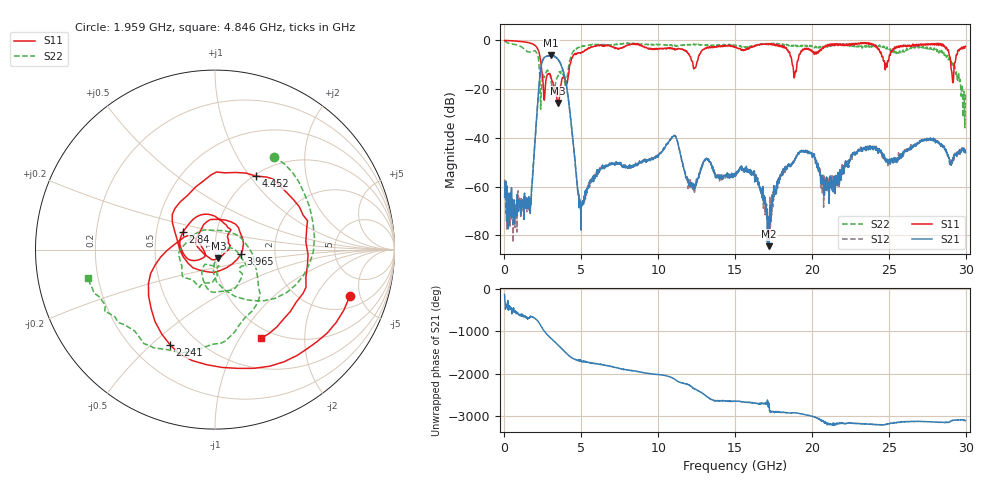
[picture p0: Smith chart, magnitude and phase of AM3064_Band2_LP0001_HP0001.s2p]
# Hz S DB R 50.0
!freq dBS11 angS11 dBS21 angS21 dBS12 angS12 dBS22 angS22
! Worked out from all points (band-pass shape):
!   1600 points, 10 MHz to 29.98 GHz, reference 50 ohm
!   highest |S21| = -6.21 dB at 3.046 GHz (marker M1); lowest = -84.5 dB at 17.22 GHz (marker M2)
!   |S21| within 3 dB of the highest: 2.436 GHz to 3.608 GHz (1.172 GHz wide, 38.8 % of centre)
!   lowest |S11| = -25.7 dB at 3.478 GHz (marker M3), VSWR 1.11, Z = 51.7 - j5.02 ohm
!   |S11| at or under -10 dB: 2.385 GHz to 4.259 GHz (1.874 GHz wide, 56.4 % of centre); 18.73 GHz to 19.02 GHz (292 MHz wide, 1.55 % of centre); 29.03 GHz to 29.26 GHz (229.2 MHz wide, 0.786 % of centre)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
!   |S22| runs from -35.9 to -0.2 dB; largest |S21 - S12| = 0.016
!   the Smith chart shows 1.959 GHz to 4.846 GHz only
!   S11 on the Smith chart (normalised r, x): 1.959 GHz: 2.90, -4.03; 2.241 GHz: 0.36, -0.57; 2.84 GHz: 0.69, +0.14; 3.965 GHz: 1.34, -0.07; 4.452 GHz: 1.02, +1.07; 4.846 GHz: 0.87, -1.24
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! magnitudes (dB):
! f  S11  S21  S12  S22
! 10 MHz  -0.1  -64.4  -57.1  -0.2
! 1.603 GHz  -1.0  -67.1  -69.7  -4.8
! 1.959 GHz  -2.0  -43.5  -43.9  -4.2
! 2.241 GHz  -4.6  -19.2  -19.2  -9.5
! 2.84 GHz  -13.8  -6.4  -6.3  -12.6
! 3.046 GHz  -15.5  -6.2  -6.2  -17.4
! 3.478 GHz  -25.7  -7.7  -7.9  -14.7
! 3.965 GHz  -16.6  -16.5  -16.5  -19.1
! 4.452 GHz  -6.6  -41.1  -40.8  -4.7
! 4.846 GHz  -5.1  -63.9  -63.5  -2.8
! 5.015 GHz  -5.1  -67.9  -67.2  -2.7
! 10 GHz  -3.4  -48.0  -47.1  -1.7
! 15 GHz  -2.6  -55.5  -55.1  -1.9
! 16.26 GHz  -2.4  -53.7  -55.0  -2.3
! 17.22 GHz  -1.3  -84.5  -76.7  -1.4
! 18.12 GHz  -2.9  -54.0  -55.3  -1.5
! 19.99 GHz  -4.2  -46.3  -47.1  -2.2
! 20.98 GHz  -2.1  -59.0  -59.6  -2.9
! 25 GHz  -8.0  -50.0  -48.9  -3.0
! 28.56 GHz  -2.1  -43.3  -43.8  -5.0
! 29.18 GHz  -17.4  -49.1  -50.1  -9.4
! 29.98 GHz  -2.4  -46.2  -45.7  -21.7
